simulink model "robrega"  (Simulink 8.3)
settings: Solver=ode5  StartTime=0.0  StopTime=15  FixedStep=10e-5  RelTol=1e-6  AbsTol=1e-6

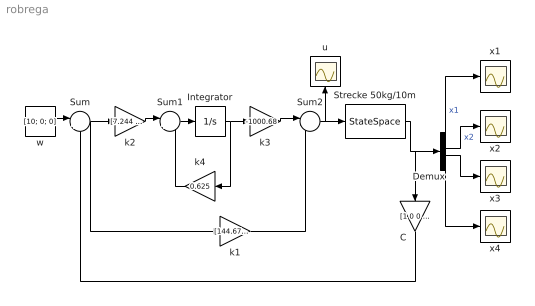
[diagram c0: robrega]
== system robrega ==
  C : Gain  Gain=[1 0 0 0;0 1 0 0;0 0 1 0]  Multiplication=Matrix(K*u)
  Demux : Demux
  Integrator : Integrator
  Strecke 50kg/10m : StateSpace  A=[0 1 0 0;0 0 0.4905 0;0 0 0 1;0 0 -1.03005 0]  B=[0;0.001;0; -0.0001]  C=[1 0 0 0;0 1 0 0;0 0 1 0;0 0 0 1]  D=[0;0;0;0]  X0=[0;0;0;0]
  Sum : Sum  Inputs=|+-
  Sum1 : Sum  Inputs=|+-
  Sum2 : Sum  Inputs=|-+
  k1 : Gain  Gain=[144.675 10294.8 -10032.5]  Multiplication=Matrix(K*u)
  k2 : Gain  Gain=[7.244 25.353 -306.174]  Multiplication=Matrix(K*u)
  k3 : Gain  Gain=-1000.68  Multiplication=Matrix(K*u)
  k4 : Gain  Gain=0.625  Multiplication=Matrix(K*u)
  u : Scope
  w : Constant  Value=[10; 0; 0]
  x{1..4} (4 alike) : Scope
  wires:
  w/1 -> Sum/1
  k2/1 -> Sum1/1
  Sum1/1 -> Integrator/1
  k3/1 -> Sum2/1
  Sum2/1 -> Strecke 50kg/10m/1, u/1
  Demux/3 -> x3/1
  Demux/4 -> x4/1
  Demux/1 -> x1/1  "x1"
  Demux/2 -> x2/1  "x2"
  Strecke 50kg/10m/1 -> Demux/1, C/1
  C/1 -> Sum/2
  Sum/1 -> k2/1, k1/1
  k1/1 -> Sum2/2
  k4/1 -> Sum1/2
  Integrator/1 -> k3/1, k4/1
